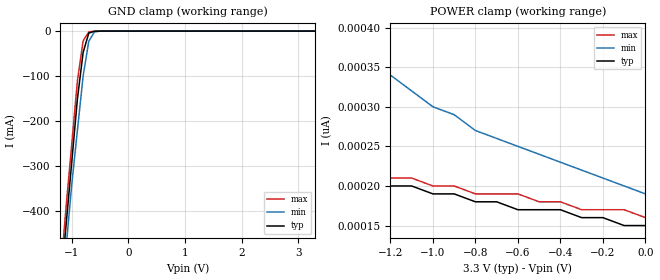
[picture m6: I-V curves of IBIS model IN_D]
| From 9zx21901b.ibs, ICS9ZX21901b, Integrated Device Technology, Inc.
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|   Model IN_D
[Model]   IN_D
Model_type   Input
Polarity   Inverting
Enable   Active-High
Vinl =   1.00V
Vinh =   2.00V
C_comp   3.40pF   2.85pF   3.95pF
[Temperature Range]   27.00   70.00   0.000
[Voltage Range]   3.30V   3.00V   3.60V
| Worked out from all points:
|   GND clamp passes 1 mA (typ) near -0.62 V on its own axis
[GND_clamp]
| voltage   I(typ)   I(min)   I(max)
-3.3V     -3.78A     -3.65A     -3.87A
-1.2V     -570mA     -610mA     -540mA
-1.1V     -430mA     -480mA     -390mA
-1V       -290mA     -340mA     -250mA
-900mV    -150mA     -220mA     -110mA
-800mV    -47.77mA   -100mA     -21.77mA
-700mV    -4.42mA    -22.5mA    -1.71mA
-600mV    -390uA     -1.83mA    -190uA
-500mV    -33.14uA   -140uA     -13.41uA
3.3V      150pA      220pA      150pA
[POWER_clamp]
| voltage   I(typ)   I(min)   I(max)
-3.3V     350pA      1.67nA     300pA
-2.6V     280pA      890pA      270pA
-2.5V     280pA      820pA      260pA
-2.3V     260pA      700pA      260pA
-2.2V     250pA      640pA      250pA
-1.5V     220pA      400pA      220pA
-1.4V     210pA      380pA      220pA
-1V       190pA      300pA      200pA
-800mV    180pA      270pA      190pA
-600mV    170pA      250pA      190pA
-400mV    170pA      230pA      180pA
0V        150pA      190pA      160pA
